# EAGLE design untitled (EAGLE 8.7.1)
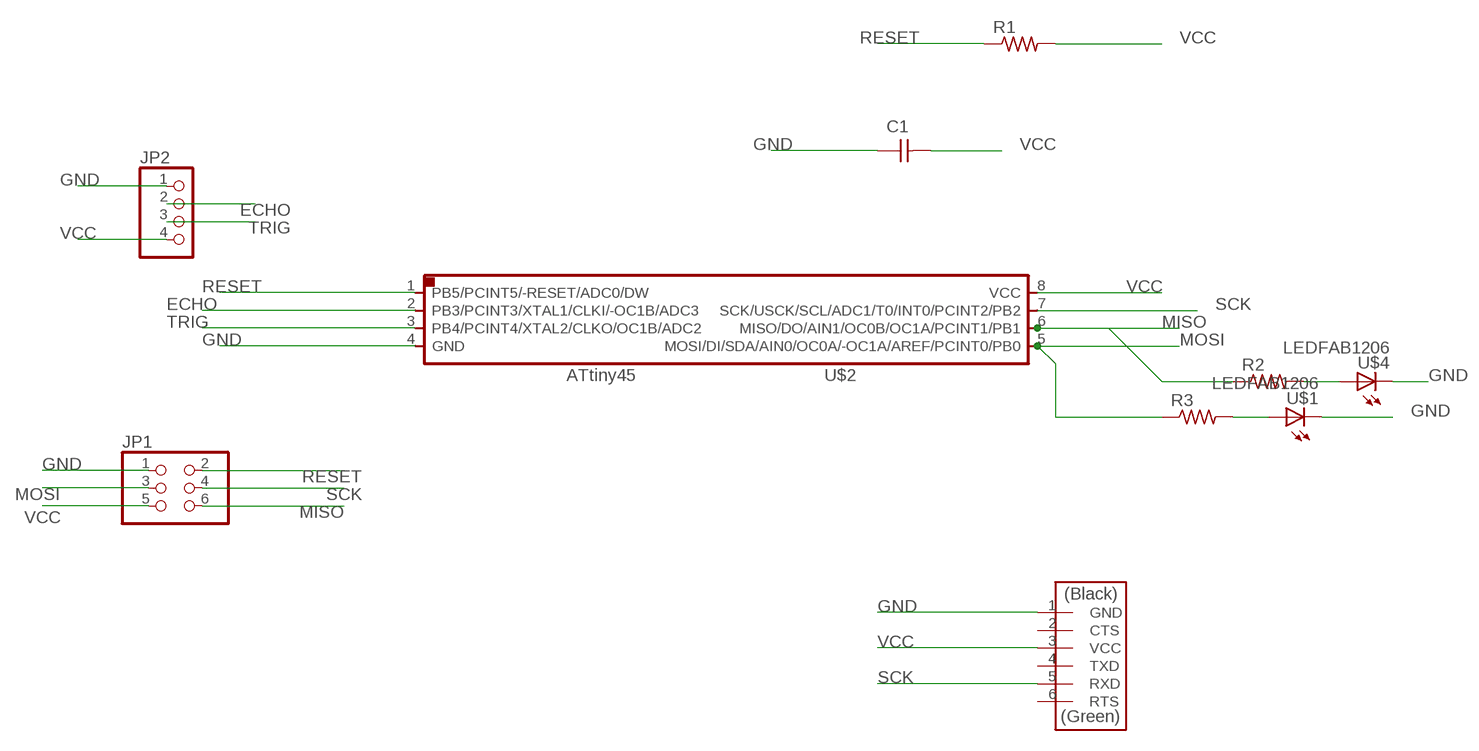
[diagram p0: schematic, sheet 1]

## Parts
C1  CAP-UNPOLARIZEDFAB  [C1206FAB]
JP1  PINHD-2X3-SMD  [2X03SMD]
JP2  PINHD-1X4  [1X04]
R1  RES-US1206FAB  [R1206FAB]
R2  RES-US1206FAB  [R1206FAB]
R3  RES-US1206FAB  [R1206FAB]
U$1  LEDFAB1206  [LED1206FAB]
U$2  ATTINY45SI  [SOIC8]
U$3  FTDI-SMD-HEADER  [1X06SMD]
U$4  LEDFAB1206  [LED1206FAB]

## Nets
ECHO: JP2.2 U$2.2(PB3/PCINT3/XTAL1/CLKI/-OC1B/ADC3)
GND: C1.1 JP1.1 JP2.1 U$1.2(C) U$2.4(GND) U$3.1(GND) U$4.2(C)
MISO: JP1.6 R2.1 U$2.6(MISO/DO/AIN1/OC0B/OC1A/PCINT1/PB1)
MOSI: JP1.3 R3.1 U$2.5(MOSI/DI/SDA/AIN0/OC0A/-OC1A/AREF/PCINT0/PB0)
N$1: R2.2 U$4.1(A)
N$2: R3.2 U$1.1(A)
RESET: JP1.2 R1.1 U$2.1(PB5/PCINT5/-RESET/ADC0/DW)
SCK: JP1.4 U$2.7(SCK/USCK/SCL/ADC1/T0/INT0/PCINT2/PB2) U$3.5(RXD)
TRIG: JP2.3 U$2.3(PB4/PCINT4/XTAL2/CLKO/OC1B/ADC2)
VCC: C1.2 JP1.5 JP2.4 R1.2 U$2.8(VCC) U$3.3(VCC)
Unconnected: U$3.2(CTS) U$3.4(TXD) U$3.6(RTS)

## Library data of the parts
C1 = fab:CAP-UNPOLARIZED
JP1 = fab:PINHD-2X3-SMD: PIN HEADER
JP2 = pinhead:PINHD-1X4: PIN HEADER
R1-R3 = fab:RES-US: Resistor (US Symbol)
U$1 U$4 = fab:LED: LED
U$2 = fab:ATTINY45
U$3 = fab:FTDI-SMD-HEADER

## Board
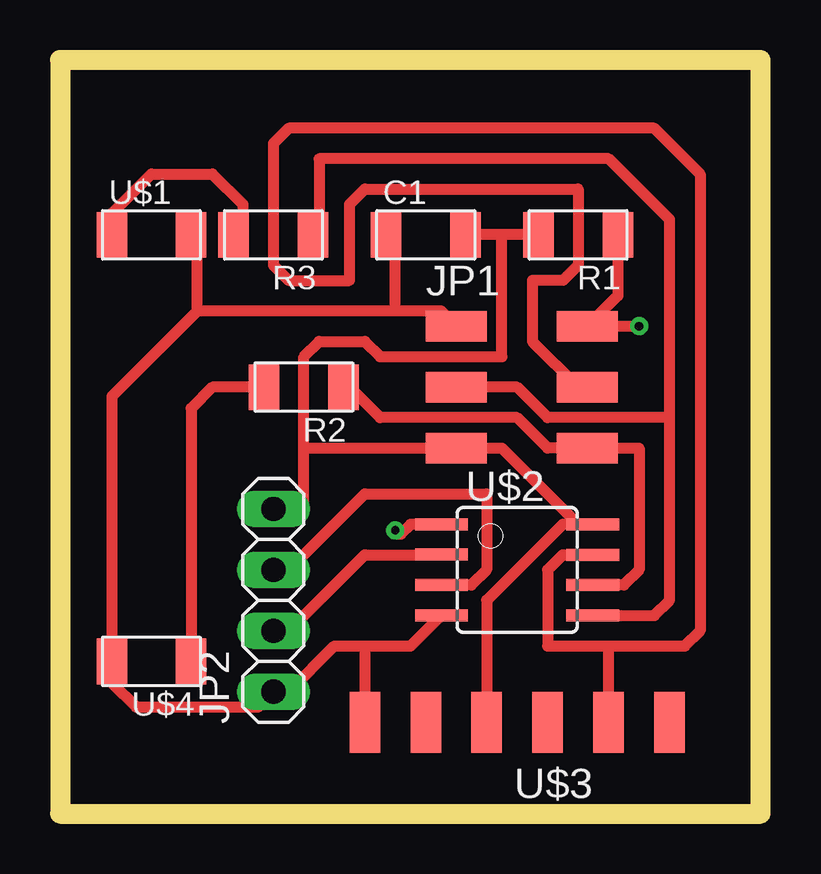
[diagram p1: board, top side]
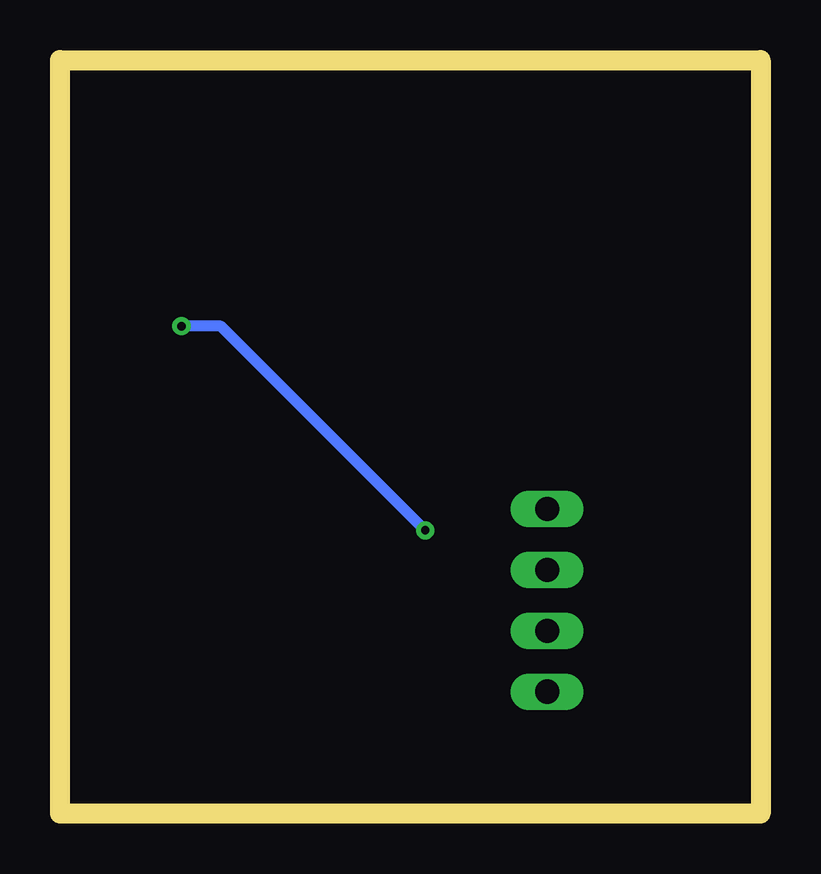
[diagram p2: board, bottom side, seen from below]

Size 29.19 x 31.42 mm. Coordinates in mm from the lower left corner, seen from the top.
Outline: 0,0 29.19,0 29.19,31.42 0,31.42 0,0
Copper layers (1*16): Top 0.035mm / dielectric 1.5mm / Bottom 0.035mm
Design rules "default *": minimum track width 18mil, minimum drill 0.35mm, track to track 16mil, track to pad 16mil, pad to pad 16mil, via to via 16mil, smd to smd 16mil, copper to edge 40mil, drill to drill 6mil, minimum pad ring 10mil, minimum via ring 8mil, stop-mask expansion 4mil, vias tented up to drill 0mil, thermal gap 10mil

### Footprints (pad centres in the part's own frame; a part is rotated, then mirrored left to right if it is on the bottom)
C1206FAB = smd 1.27 x 1.905: 1 -1.651,0; 2 1.651,0
2X03SMD = smd 2.54 x 1.27: 1 -2.54,2.54; 2 2.92,2.54; 3 -2.54,0; 4 2.92,0; 5 -2.54,-2.54; 6 2.92,-2.54
1X04 = drill 1.016 long: 1 -3.81,0; 2 -1.27,0; 3 1.27,0; 4 3.81,0
R1206FAB = smd 1.27 x 1.905: 1 -1.651,0; 2 1.651,0
LED1206FAB = smd 1.27 x 1.905: 1 -1.651,0; 2 1.651,0
SOIC8 = smd 0.5 x 2.2: 1 -1.905,-3.154; 2 -0.645,-3.154; 3 0.625,-3.154; 4 1.895,-3.154; 5 1.905,3.154; 6 0.635,3.154; 7 -0.635,3.154; 8 -1.905,3.154
1X06SMD = smd 2.54 x 1.27: 1 0,6.35; 2 0,3.81; 3 0,1.27; 4 0,-1.27; 5 0,-3.81; 6 0,-6.35

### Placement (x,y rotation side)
C1  15.24,24.13 0 top
JP1  19.05,17.78 0 top
JP2  8.89,8.89 90 top
R1  21.59,24.13 180 top
R2  10.16,17.78 180 top
R3  8.89,24.13 180 top
U$1  3.81,24.13 0 top
U$2  19.05,10.16 270 top
U$3  19.05,3.81 90 top
U$4  3.81,6.35 180 top

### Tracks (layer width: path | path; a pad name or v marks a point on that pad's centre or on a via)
ECHO
  Top 0.457: JP2.2 9.52,7.62 12.7,10.8 15.88,10.8 U$2.2
GND
  Top 0.457: 5.72,20.95 5.72,24.13 U$1.2 | 13.97,20.95 15.88,20.95 JP1.1 | 13.97,20.95 5.72,20.95 | 13.97,20.95 13.97,24.13 C1.1 | 12.7,6.99 11.43,6.99 9.52,5.08 JP2.1 8.25,4.45 3.17,4.45 2.16,5.46 U$4.2 2.16,17.4 5.72,20.95 | 12.7,6.99 14.61,6.99 15.88,8.25 U$2.4 | 12.7,6.99 U$3.1
MISO
  Top 0.457: R2.1 12.06,17.78 13.33,16.51 19.05,16.51 20.32,15.24 JP1.6 24.13,15.24 24.13,10.16 23.49,9.53 U$2.6
MOSI
  Top 0.457: 25.4,16.51 25.4,24.77 22.86,27.3 10.79,27.3 10.79,24.13 R3.1 | JP1.3 19.05,17.78 20.32,16.51 25.4,16.51 | 25.4,16.51 25.4,8.89 24.76,8.25 U$2.5
N$1
  Top 0.457: R2.2 6.35,17.78 5.46,16.89 U$4.1
N$2
  Top 0.457: U$1.1 2.16,25.02 3.81,26.67 6.35,26.67 7.62,25.4 7.62,24.51 R3.2
RESET  (via drill 0.35)
  Top 0.457: R1.1 23.24,21.59 JP1.2 v24.13,20.32 | U$2.1 14.61,12.07 14.2,11.66 | 13.97,11.66 14.2,11.66 | 14.2,11.66 14.05,11.81 v13.97,11.81
  Bottom 0.457: v13.97,11.81 22.48,20.32 v24.13,20.32
SCK
  Top 0.457: U$2.7 20.95,10.8 20.32,10.16 20.32,6.99 22.86,6.99 | 22.86,5.71 U$3.5 22.86,6.99 | JP1.4 21.59,17.78 19.68,19.68 19.68,22.22 20.95,22.22 21.59,22.86 21.59,26.04 12.7,26.04 12.06,25.4 12.06,22.22 9.52,22.22 8.89,22.86 8.89,27.94 9.52,28.57 24.76,28.57 26.67,26.67 26.67,7.62 26.04,6.99 22.86,6.99
TRIG
  Top 0.457: JP2.3 9.52,10.16 12.7,13.34 17.78,13.34 17.78,10.16 17.14,9.53 16.51,9.53 U$2.3
VCC
  Top 0.457: 21.59,12.07 18.41,15.24 JP1.5 10.16,15.24 | U$3.3 17.78,8.89 20.95,12.07 21.59,12.07 | 21.59,12.07 U$2.8 | R1.2 18.41,24.13 | 18.41,24.13 C1.2 | 18.41,24.13 18.41,19.05 13.33,19.05 12.7,19.68 10.79,19.68 10.16,19.05 10.16,15.24 | 10.16,15.24 10.16,12.7 JP2.4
